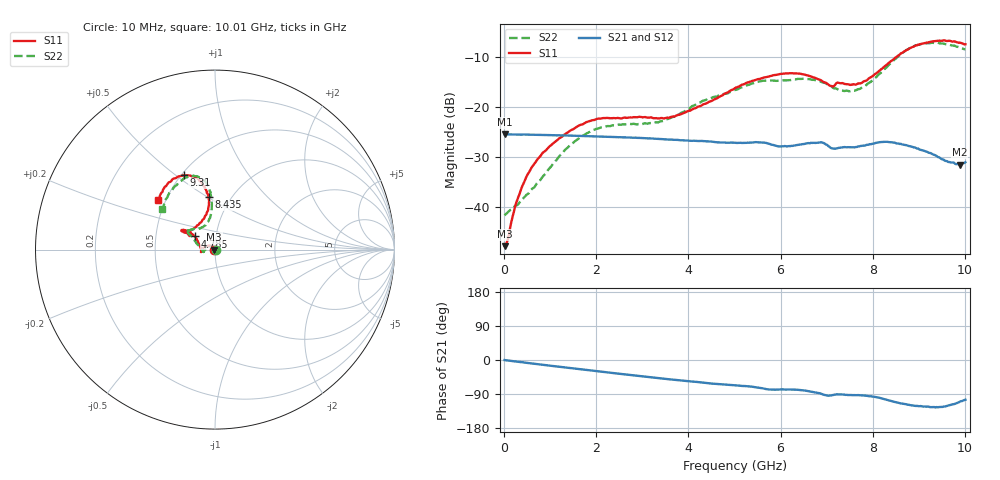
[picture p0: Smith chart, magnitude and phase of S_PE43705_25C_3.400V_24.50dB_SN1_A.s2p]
! Device ID: PE43705
! Serial: 1
! Insertion: A
! Impedance: 50 ohm
! Temp: 25C
! VDD: 3.400V
! Attenuation Step: 24.50dB
#  Hz  S  RI  R  50
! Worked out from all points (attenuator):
!   401 points, 10 MHz to 10.01 GHz, reference 50 ohm
!   highest |S21| = -25.50 dB at 10 MHz (marker M1); lowest = -31.5 dB at 9.885 GHz (marker M2)
!   lowest |S11| = -47.8 dB at 10 MHz (marker M3), VSWR 1.01, Z = 49.6 + j0.0428 ohm
!   |S11| at or under -10 dB: start of sweep to 8.522 GHz
!   |S22| runs from -41.7 to -7.2 dB; largest |S21 - S12| = 0.00073
!   S11 on the Smith chart (normalised r, x): 10 MHz: 0.99, +0.00; 4.785 GHz: 0.79, +0.12; 8.435 GHz: 0.79, +0.50; 9.31 GHz: 0.51, +0.53; 10.01 GHz: 0.46, +0.31
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1e7  -0.00404 0.000431  0.0531 -0.000218  0.0531 -0.0002  0.00822 0.000294
8.5e7  -0.0038 0.00301  0.0529 -0.00129  0.0529 -0.00124  0.00861 0.00234
3.1e8  -0.00637 0.0109  0.0526 -0.00441  0.0526 -0.00438  0.0061 0.00881
5.85e8  -0.0148 0.0192  0.0519 -0.00809  0.0519 -0.00804  -0.0014 0.0147
1.01e9  -0.035 0.0215  0.0503 -0.0136  0.0503 -0.0136  -0.0204 0.0145
1.685e9  -0.0659 0.00864  0.0464 -0.0215  0.0465 -0.0215  -0.0508 0.00197
2.21e9  -0.0769 -0.00752  0.0425 -0.0268  0.0425 -0.0268  -0.0627 -0.0103
3.36e9  -0.0761 -0.00547  0.0317 -0.0356  0.0318 -0.0355  -0.0703 -0.00176
3.86e9  -0.0831 0.019  0.0271 -0.0376  0.0269 -0.0377  -0.0858 0.0173
4.785e9  -0.1131 0.0735  0.0188 -0.0398  0.0188 -0.0396  -0.1197 0.0618
5.01e9  -0.1265 0.0865  0.0172 -0.0402  0.0172 -0.0401  -0.1284 0.0712
5.985e9  -0.1812 0.1098  0.0086 -0.0394  0.00882 -0.0393  -0.1501 0.102
6.685e9  -0.1733 0.0961  0.0045 -0.0433  0.00444 -0.0433  -0.1516 0.1066
7.11e9  -0.1387 0.0802  -0.00205 -0.0384  -0.00195 -0.0384  -0.1105 0.1139
7.585e9  -0.1003 0.1343  -0.00177 -0.0393  -0.00167 -0.0393  -0.0586 0.1323
7.91e9  -0.0572 0.182  -0.00384 -0.0416  -0.00368 -0.0419  -0.0328 0.1688
8.36e9  -0.0331 0.274  -0.0129 -0.0424  -0.0125 -0.0425  -0.0184 0.2638
8.435e9  -0.0356 0.2912  -0.0145 -0.0415  -0.0143 -0.0415  -0.0196 0.2833
8.86e9  -0.0871 0.3842  -0.0197 -0.0346  -0.0194 -0.0344  -0.0668 0.3886
9.31e9  -0.1754 0.4138  -0.0189 -0.0275  -0.0187 -0.0275  -0.1489 0.4072
9.885e9  -0.2989 0.3165  -0.00924 -0.0248  -0.00945 -0.0251  -0.275 0.2793
1.001e10  -0.3157 0.2759  -0.00718 -0.027  -0.00689 -0.0274  -0.2954 0.2288
